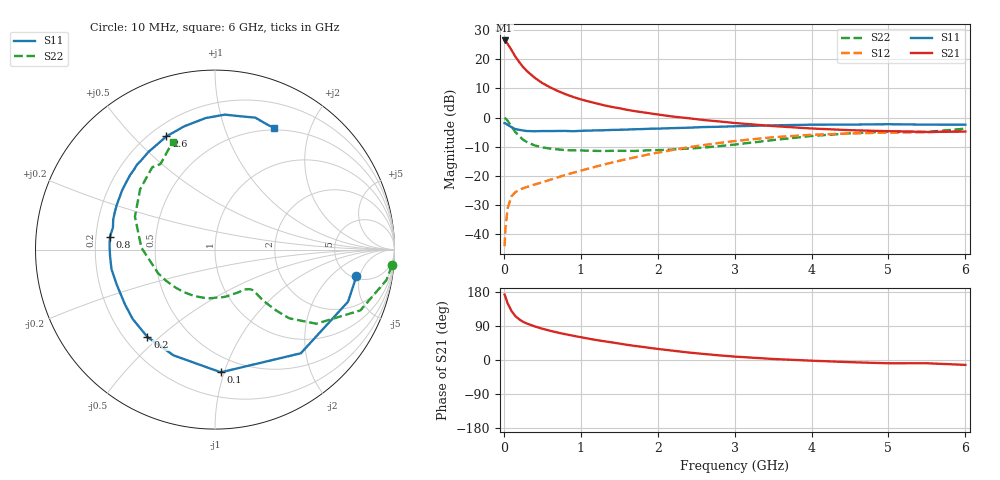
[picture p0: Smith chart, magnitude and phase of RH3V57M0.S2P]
! SIEMENS Small Signal Semiconductors
! BFR106
! Si NPN RF Bipolar Junction Transistor in SOT23
! VCE = 3.5 V  IC = 7 mA
! Common Emitter S-Parameters:  August  1996
# GHz  S  MA  R  50
!  f  S11  S21  S12  S22
! GHz  MAG  ANG  MAG  ANG  MAG  ANG  MAG  ANG
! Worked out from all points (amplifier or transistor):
!   36 points, 10 MHz to 6 GHz, reference 50 ohm
!   highest |S21| = 26.5 dB at 10 MHz (marker M1)
!   |S21| within 3 dB of that: start of sweep to 92.49 MHz
!   unconditionally stable (mu >= 1): 556.9 MHz to 2.071 GHz; 4.958 GHz to end of sweep
!   at 250 MHz: K = 0.60, MSG = 20.8 dB, |S12| = -24.3 dB
!   at 1.4 GHz: K = 1.12, MAG = 7.5 dB, |S12| = -15.5 dB
!   at 6 GHz: K = 1.02, MAG = -0.9 dB, |S12| = -4.6 dB
!   S11 on the Smith chart (normalised r, x): 10 MHz: 5.32, -4.44; 100 MHz: 0.38, -0.97; 200 MHz: 0.29, -0.46; 800 MHz: 0.26, +0.06; 2.6 GHz: 0.26, +0.63; 6 GHz: 0.48, +1.49
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0.01  0.8021 -10.7  21.04 172.7  0.0062 86.3  0.9895 -5.1
0.02  0.796 -21.4  20.58 167.0  0.0124 80.7  0.9708 -10.0
0.05  0.7498 -50.4  18.36 149.2  0.0279 65.6  0.8781 -22.7
0.1  0.6844 -87.3  14.36 129.3  0.0446 52.0  0.6992 -36.2
0.15  0.6329 -111.4  11.08 115.7  0.0524 44.9  0.5634 -42.8
0.2  0.6154 -127.7  8.96 107.4  0.0576 42.6  0.4794 -44.9
0.25  0.5999 -139.8  7.388 100.7  0.0612 41.6  0.4169 -46.1
0.3  0.5875 -148.5  6.278 96.2  0.0643 42.4  0.3803 -46.7
0.4  0.5814 -160.7  4.834 88.8  0.0709 44.6  0.3326 -46.7
0.5  0.5869 -169.2  3.911 82.6  0.0774 47.6  0.3073 -47.1
0.6  0.5859 -176.5  3.306 77.2  0.0854 50.5  0.2935 -48.7
0.8  0.5896 172.9  2.52 68.0  0.1034 54.6  0.2766 -53.4
0.9  0.5819 167.8  2.257 64.1  0.1127 56.5  0.2731 -55.6
1.1  0.5965 159.1  1.891 56.4  0.1331 58.9  0.2701 -63.0
1.3  0.6054 151.7  1.625 49.6  0.1561 60.0  0.2668 -70.7
1.6  0.622 142.2  1.359 40.1  0.1941 60.1  0.2681 -84.0
2.2  0.6585 124.3  1.039 24.5  0.2791 55.6  0.2832 -113.9
2.6  0.6869 113.2  0.906 15.9  0.3376 50.1  0.3051 -136.1
3.5  0.7347 94.1  0.714 2.7  0.4592 34.7  0.4102 178.5
4.5  0.7564 79.0  0.607 -5.7  0.5331 16.4  0.536 141.1
5.5  0.7556 67.7  0.566 -8.6  0.5602 5.0  0.5653 122.5
6  0.7533 64.0  0.575 -12.9  0.5896 -2.8  0.6454 111.4
